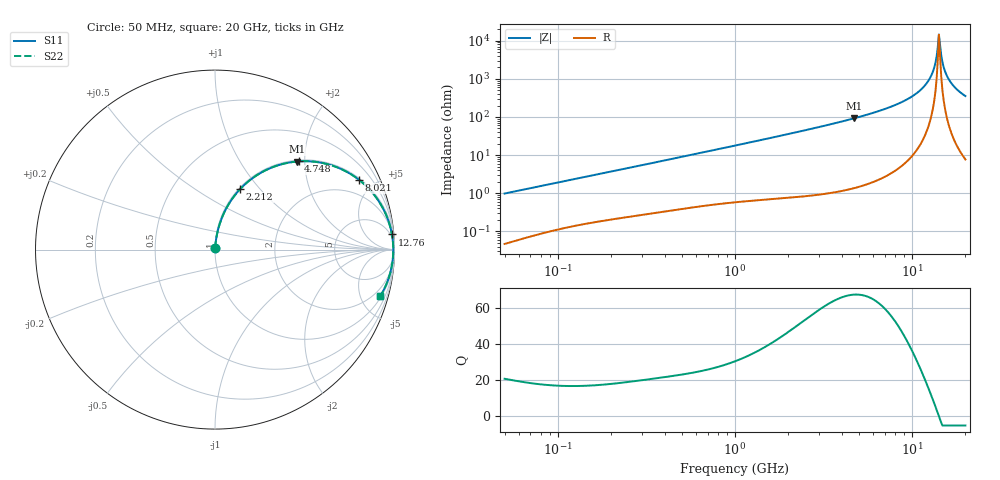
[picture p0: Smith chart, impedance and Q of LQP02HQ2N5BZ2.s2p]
!Murata Part Number: LQP02HQ2N5BZ2
!These Parameters are Measured in Series Mode Connection
!  o--[Z]--o
!Port1  Port2
!  o-------o
!Freq. Start=50[MHz] Stop=20[GHz], 401[Steps]
# Hz S RI R 50
!Freq.(Hz) S11(Real) S11(Imag) S21(Real) S21(Imag) S12(Real) S12(Imag) S22(Real) S22(Imag)
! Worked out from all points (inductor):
!   401 points, 50 MHz to 20 GHz, reference 50 ohm
!   read as one part in series: L = 3.11 nH near 51.52 MHz
!   highest Q = 67.6 at 4.678 GHz (marker M1), where L = 3.12 nH
!   self-resonance near 14.17 GHz
!   S11 on the Smith chart (normalised r, x): 50 MHz: 1.00, +0.02; 2.212 GHz: 1.02, +0.79; 4.748 GHz: 1.03, +1.87; 8.021 GHz: 1.08, +4.11; 12.76 GHz: 3, +23; 20 GHz: 1.15, -7.08
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5e7  0.000568 0.00985  0.9994 -0.00985  0.9994 -0.00985  0.000568 0.00985
1.364002e8  0.00218 0.0257  0.9978 -0.0257  0.9978 -0.0257  0.00218 0.0257
3.721004e8  0.00766 0.0669  0.9923 -0.0669  0.9923 -0.0669  0.00766 0.0669
1e9  0.0359 0.1704  0.9641 -0.1704  0.9641 -0.1704  0.0359 0.1704
2.211938e9  0.141 0.3382  0.859 -0.3382  0.859 -0.3382  0.141 0.3382
2.728004e9  0.2012 0.3921  0.7988 -0.3921  0.7988 -0.3921  0.2012 0.3921
4.677679e9  0.4568 0.4908  0.5432 -0.4908  0.5432 -0.4908  0.4568 0.4908
4.748272e9  0.466 0.4915  0.534 -0.4915  0.534 -0.4915  0.466 0.4915
7.442007e9  0.7583 0.4194  0.2417 -0.4194  0.2417 -0.4194  0.7583 0.4194
8.020766e9  0.804 0.3876  0.196 -0.3876  0.196 -0.3876  0.804 0.3876
1.082228e10  0.9466 0.2084  0.0534 -0.2084  0.0534 -0.2084  0.9466 0.2084
1.183995e10  0.972 0.1422  0.028 -0.1422  0.028 -0.1422  0.972 0.1422
1.276073e10  0.9858 0.0844  0.0142 -0.0844  0.0142 -0.0844  0.9858 0.0844
1.334722e10  0.9907 0.0489  0.00927 -0.0489  0.00927 -0.0489  0.9907 0.0489
1.375312e10  0.9926 0.0251  0.00742 -0.0251  0.00742 -0.0251  0.9926 0.0251
1.417136e10  0.9933 0.00128  0.00671 -0.00128  0.00671 -0.00128  0.9933 0.00128
1.460232e10  0.9928 -0.0226  0.00716 0.0226  0.00716 0.0226  0.9928 -0.0226
1.504638e10  0.9912 -0.0464  0.00875 0.0464  0.00875 0.0464  0.9912 -0.0464
1.527346e10  0.99 -0.0583  0.00998 0.0583  0.00998 0.0583  0.99 -0.0583
1.597544e10  0.9846 -0.0937  0.0154 0.0937  0.0154 0.0937  0.9846 -0.0937
1.747767e10  0.9663 -0.1626  0.0337 0.1626  0.0337 0.1626  0.9663 -0.1626
2e10  0.9212 -0.2587  0.0788 0.2587  0.0788 0.2587  0.9212 -0.2587
